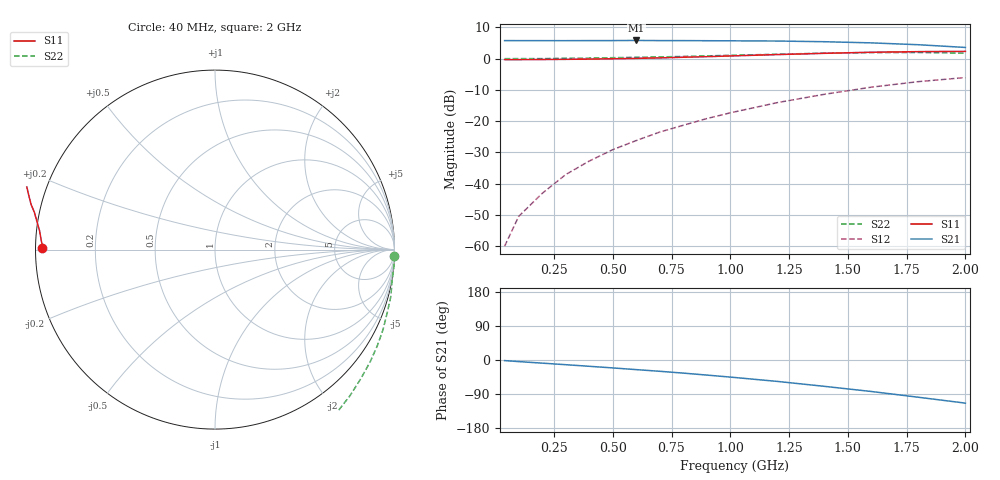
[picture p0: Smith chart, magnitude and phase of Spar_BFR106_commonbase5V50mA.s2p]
! Filename:  BFR106CC.S2P  Version:  2.0
! NXP part #: BFR106  Date: Jul 1990
! Bias condition: Vce=5V, Ic=50mA
! COMMON BASE
#  MHz  S  MA  R  50
! Freq  S11  S21  S12  S22
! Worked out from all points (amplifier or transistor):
!   16 points, 40 MHz to 2 GHz, reference 50 ohm
!   highest |S21| = 5.8 dB at 600 MHz (marker M1)
!   |S21| within 3 dB of that: start of sweep to end of sweep
!   unconditionally stable (mu >= 1): nowhere
!   at 200 MHz: K = -0.53, MSG = 24.4 dB, |S12| = -43.1 dB
!   at 800 MHz: K = -0.93, MSG = 13.5 dB, |S12| = -21.3 dB
!   at 2 GHz: K = -0.84, MSG = 4.8 dB, |S12| = -6.0 dB
40  0.965 179.5  1.945 -1.6  0.001 66.1  1 -1.9
100  0.964 178.2  1.944 -4.2  0.003 106.5  1.002 -5.0
200  0.97 176.9  1.942 -8.3  0.007 118.1  1.002 -9.9
300  0.976 175.4  1.941 -12.4  0.014 131.5  1.014 -15.0
400  0.984 173.7  1.946 -16.6  0.023 135.8  1.022 -20.1
500  0.997 172.0  1.947 -20.9  0.035 138.7  1.037 -25.5
600  1.011 170.2  1.956 -25.4  0.049 138.9  1.051 -30.6
700  1.029 168.2  1.946 -29.8  0.067 139.0  1.067 -35.9
800  1.054 166.3  1.945 -34.6  0.086 138.9  1.085 -41.5
900  1.077 164.1  1.937 -39.8  0.11 136.5  1.108 -47.2
1000  1.105 161.6  1.931 -45.1  0.136 134.0  1.132 -52.9
1200  1.163 156.2  1.915 -56.5  0.198 128.5  1.177 -65.3
1400  1.218 149.7  1.867 -69.5  0.269 120.9  1.226 -78.4
1600  1.267 142.4  1.789 -83.1  0.35 113.1  1.25 -92.0
1800  1.295 134.0  1.671 -98.3  0.429 103.7  1.256 -106.6
2000  1.309 126.5  1.512 -113.8  0.499 94.5  1.225 -121.0
